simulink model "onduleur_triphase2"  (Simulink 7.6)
settings: Solver=FixedStepDiscrete  StartTime=0.0  StopTime=0.004  RelTol=1e-3
InitFcn:
  | clc
  | close all
  | clear all
  | Ts=5e-5;
undefined symbols (not defined in the file or in its folder): arm, bridge, pulses
libraries: powerlib x9, powerlib_extras x1

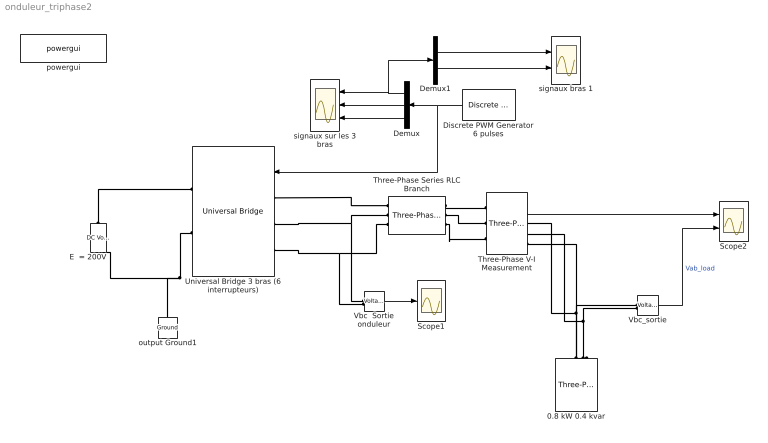
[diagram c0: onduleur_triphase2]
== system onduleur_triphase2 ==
  0.8 kW 0.4 kvar : powerlib/Elements/Three-Phase Parallel RLC Load  DialogController=POWERSYS.PowerSysDialog  PhysicalDomain=powersysdomain  SubClassName=unknown  LeftPortType=p1  RightPortType=p1  LConnTagsString=A|B|C  Configuration=Y (grounded)  NominalVoltage=140  NominalFrequency=60  ActivePower=800  InductivePower=0  CapacitivePower=400  Measurements=None
  Demux : Demux  Outputs=3
  Demux1 : Demux  Outputs=2
  Discrete PWM Generator 6 pulses : powerlib_extras/Discrete  Control Blocks/Discrete PWM Generator  DialogController=POWERSYS.PowerSysDialog  SystemSampleTime=-1  GeneratorMode="3-arm  bridge (6 pulses)"  Fc=1080  Ts=Ts  Internal=on  mIndex=0.8  Freq=60  Phase=0
  E  = 200V : powerlib/Electrical Sources/DC Voltage Source  Description=source block  DialogController=POWERSYS.PowerSysDialog  SystemSampleTime=-1  Amplitude=200  Measurements=None
  Scope1 : Scope
  Scope2 : Scope  NumInputPorts=2
  Three-Phase Series RLC Branch : powerlib/Elements/Three-Phase Series RLC Branch  DialogController=POWERSYS.PowerSysDialog  PhysicalDomain=powersysdomain  SubClassName=unknown  LeftPortType=p1  RightPortType=p1  LConnTagsString=A|B|C  RConnTagsString=A|B|C  BranchType=RL  Resistance=4  Inductance=1e-3  Capacitance=1e-6  Measurements=None
  Three-Phase V-I Measurement : powerlib/Measurements/Three-Phase V-I Measurement  DialogController=POWERSYS.PowerSysDialog  SystemSampleTime=-1  VoltageMeasurement=phase-to-ground  SetLabelV=off  LabelV=Vabc  Vpu=off  VpuLL=off  CurrentMeasurement=yes  SetLabelI=off  LabelI=Iabc  Ipu=off  Pbase=100e6  Vbase=500e3  OutputType=Complex  PhasorSimulation=off  PSBequivalent=0
  Universal Bridge 3 bras (6 interrupteurs) : powerlib/Power Electronics/Universal Bridge  DialogController=POWERSYS.PowerSysDialog  SystemSampleTime=-1  Arms=3  SnubberResistance=10000  SnubberCapacitance=inf  Device=IGBT / Diodes  Ron=1e-4  Lon=0  ForwardVoltages="[  1  1  ]"  ForwardVoltage=.8  GTOparameters=[ 10e-6 , 20e-6 ]  IGBTparameters=[ 1e-6 , 2e-6 ]  Measurements=None  Measurements_2=None  converterType=Rectifier
  Vbc  Sortie onduleur : powerlib/Measurements/Voltage Measurement  Tag=PoWeRsYsTeMmEaSuReMeNt  DialogController=POWERSYS.PowerSysDialog  SystemSampleTime=-1  PhasorSimulation=off  OutputType=Magnitude  PSBequivalent=0
  Vbc_sortie : powerlib/Measurements/Voltage Measurement  Tag=PoWeRsYsTeMmEaSuReMeNt  DialogController=POWERSYS.PowerSysDialog  SystemSampleTime=-1  PhasorSimulation=off  OutputType=Magnitude  PSBequivalent=0
  output Ground1 : powerlib/Elements/Ground  DialogController=POWERSYS.PowerSysDialog  PhysicalDomain=powersysdomain  SubClassName=unknown  LeftPortType=p1  RightPortType=p1  LConnTagsString=a
  powergui : powerlib/powergui  Priority=2  SystemSampleTime=-1  SimulationMode=Discrete  SampleTime=Ts  frequency=60  SPID=off  DisableSnubberDevices=off  DisableRonSwitches=off  DisableVfSwitches=off  SwTol=0  Interpol=off  frequencyindice=0  echomessages=on  HookPort=off  DisplayEquations=off  FunctionMessages=off  EnableUseOfTLC=off  x0status=blocks  RestoreLinks=warning  ResistiveCurrentMeasurement=off  Frange=[0:2:500]  Ylog=off  Xlog=off  ShowGrid=off  save=off  variable=ZData  structure=psb3phPWM1_str  ZoomFFT=on  StartTime=0.1 - 2/60  cycles=2  DisplayStyle=off  fundamental=60  FreqAxis=off  MaxFrequency=5000  frequencyindicesteady=1  RmsSteady=1  display=off  Ts=0  methode=off
  signaux bras 1 : Scope  NumInputPorts=2
  signaux sur les 3 bras : Scope  NumInputPorts=3
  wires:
  Vbc_sortie/1 -> Scope2/2  "Vab_load"
  Three-Phase V-I Measurement/2 -> Scope2/1
  Vbc  Sortie onduleur/1 -> Scope1/1
  Discrete PWM Generator 6 pulses/1 -> Demux/1, Universal Bridge 3 bras (6 interrupteurs)/1
  Demux/1 -> signaux sur les 3 bras/1, Demux1/1
  Demux/2 -> signaux sur les 3 bras/2
  Demux/3 -> signaux sur les 3 bras/3
  Demux1/2 -> signaux bras 1/2
  Demux1/1 -> signaux bras 1/1
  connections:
  0.8 kW 0.4 kvar/LConn1 -- Vbc_sortie/LConn1 -- Three-Phase V-I Measurement/RConn1
  0.8 kW 0.4 kvar/LConn2 -- Vbc_sortie/LConn2 -- Three-Phase V-I Measurement/RConn2
  Universal Bridge 3 bras (6 interrupteurs)/RConn2 -- output Ground1/LConn1 -- E  = 200V/LConn1
  E  = 200V/RConn1 -- Universal Bridge 3 bras (6 interrupteurs)/RConn1
  Three-Phase Series RLC Branch/RConn1 -- Three-Phase V-I Measurement/LConn1
  Three-Phase Series RLC Branch/RConn2 -- Three-Phase V-I Measurement/LConn2
  Three-Phase Series RLC Branch/RConn3 -- Three-Phase V-I Measurement/LConn3
  Three-Phase Series RLC Branch/LConn1 -- Universal Bridge 3 bras (6 interrupteurs)/LConn1
  Three-Phase Series RLC Branch/LConn2 -- Universal Bridge 3 bras (6 interrupteurs)/LConn2 -- Vbc  Sortie onduleur/LConn1
  Three-Phase Series RLC Branch/LConn3 -- Universal Bridge 3 bras (6 interrupteurs)/LConn3 -- Vbc  Sortie onduleur/LConn2
  Three-Phase V-I Measurement/RConn3 -- 0.8 kW 0.4 kvar/LConn3
